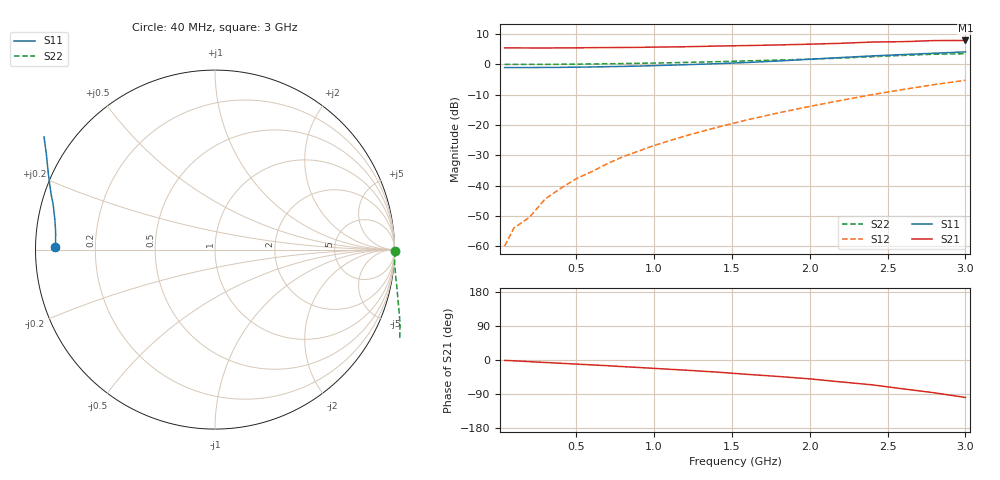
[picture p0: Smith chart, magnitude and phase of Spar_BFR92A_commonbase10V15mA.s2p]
! Filename:  BFR92ACI.S2P  Version:  2.0
! NXP part #: BFR92A  Date: Jul 1990
! Bias condition: Vce=10V, Ic=15mA
! COMMON BASE
#  MHz  S  MA  R  50
! Freq  S11  S21  S12  S22
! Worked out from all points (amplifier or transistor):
!   21 points, 40 MHz to 3 GHz, reference 50 ohm
!   highest |S21| = 7.9 dB at 3 GHz (marker M1)
!   |S21| within 3 dB of that: start of sweep to end of sweep
!   unconditionally stable (mu >= 1): nowhere
!   at 300 MHz: K = -0.59, MSG = 24.9 dB, |S12| = -44.4 dB
!   at 1 GHz: K = -0.94, MSG = 16.2 dB, |S12| = -26.7 dB
!   at 3 GHz: K = -0.89, MSG = 6.6 dB, |S12| = -5.2 dB
40  0.89 179.0  1.879 -1.0  0.001 61.3  1.002 -0.6
100  0.889 178.0  1.876 -2.1  0.002 78.0  1.004 -1.3
200  0.89 176.1  1.874 -4.4  0.003 111.8  1.003 -2.9
300  0.892 174.4  1.872 -6.5  0.006 123.9  1.003 -4.3
400  0.896 172.7  1.877 -8.6  0.009 131.5  1.008 -5.8
500  0.902 170.9  1.882 -10.8  0.013 135.1  1.013 -7.2
600  0.909 169.1  1.894 -12.9  0.017 138.9  1.019 -8.7
700  0.919 167.3  1.9 -15.0  0.023 142.7  1.026 -10.1
800  0.929 165.5  1.908 -17.5  0.03 143.7  1.035 -11.7
900  0.941 163.8  1.916 -19.7  0.037 145.6  1.044 -13.3
1000  0.957 162.1  1.934 -22.1  0.046 146.5  1.054 -14.9
1200  0.99 158.5  1.961 -26.8  0.066 147.5  1.08 -18.3
1400  1.029 154.7  2.013 -31.8  0.091 146.7  1.111 -21.9
1600  1.078 150.6  2.051 -37.9  0.122 145.8  1.145 -26.0
1800  1.141 146.6  2.101 -43.5  0.159 143.6  1.182 -30.6
2000  1.22 142.2  2.163 -49.8  0.203 140.8  1.222 -36.0
2200  1.301 137.7  2.235 -57.8  0.255 137.6  1.275 -42.4
2400  1.385 132.7  2.344 -65.5  0.317 133.2  1.342 -49.6
2600  1.457 126.2  2.379 -76.2  0.386 128.4  1.413 -57.4
2800  1.533 117.8  2.48 -86.5  0.465 121.9  1.476 -65.5
3000  1.614 108.8  2.491 -98.9  0.548 115.1  1.508 -74.8
